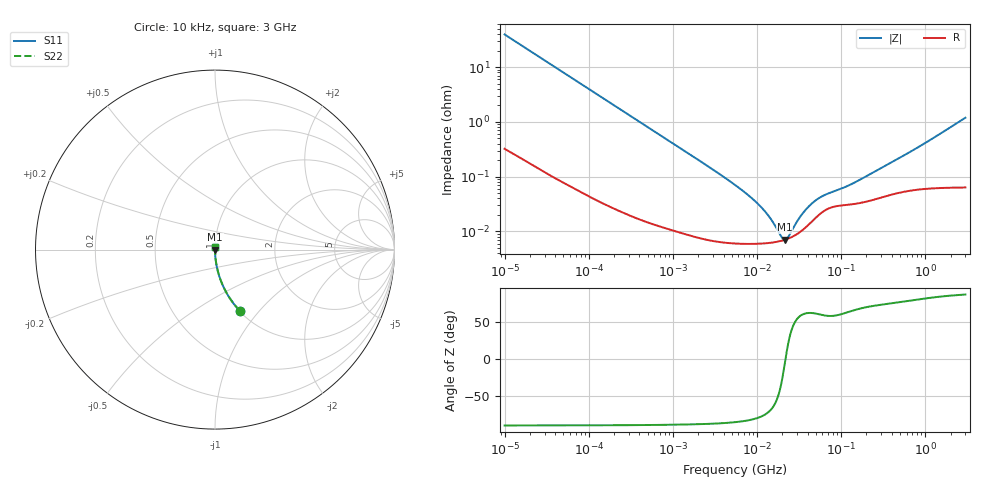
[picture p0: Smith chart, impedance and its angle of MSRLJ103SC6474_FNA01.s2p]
! MSRLJ103SC6474_FNA01  S-PARAMETER MODEL  ( Standard Model )
! Model Generated by TAIYO YUDEN Corporation (http://www.ty-top.com)
! Version 1.0
! TAIYO YUDEN Control No. 220601
! Copyright(c) 2010 TAIYO YUDEN CO.,LTD. All Rights Reserved.
! Product Description (link to TY-COMPAS)
! https://ds.yuden.co.jp/TYCOMPAS/or/detail?pn=MSRLJ103SC6474MFNA01&u=M
! Products Name : Multilayer Ceramic Capacitors
! Characteristics :
!  Capacitance : 0.47 [uF] , Rated Voltage : 6.3 [V] , TCC : X6S
!  Case Size : 0.52 x 1.0 / 0.02 x 0.039 [mm/inch] , Thickness : 0.3 / 0.012 [mm/inch]
!  (Conditions: Temperature = 25 [degC] , DC Bias Voltage = 0 [V])
! External Node Assignments :
!  1  o---| |---o  2
! GND o---------o GND
! Frequency Range : 10kHz  -  3GHz  [ 401 STEP ]
# MHZ S RI R 50
! Freq[MHz].  S11 Real  S11 Imag  S21 Real  S21 Imag  S12 Real  S12 Imag  S22 Real  S22 Imag
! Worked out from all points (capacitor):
!   401 points, 10 kHz to 3 GHz, reference 50 ohm
!   read as one part in series: C = 403 nF near 10.65 kHz
!   lowest |Z| = 7.06 mohm at 21.25 MHz (marker M1)
!   series resonance near 21.82 MHz, so ESL is about 130 pH
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0.01  0.1366 -0.3393  0.8634 0.3393  0.8634 0.3393  0.1366 -0.3393
0.016047  0.059 -0.2313  0.941 0.2313  0.941 0.2313  0.059 -0.2313
0.027426  0.0217 -0.1412  0.9783 0.1412  0.9783 0.1412  0.0217 -0.1412
0.082683  0.00283 -0.0481  0.9972 0.0481  0.9972 0.0481  0.00283 -0.0481
0.683653  0.000159 -0.00591  0.9998 0.00591  0.9998 0.00591  0.000159 -0.00591
2.652321  7.14e-05 -0.00152  0.9999 0.00152  0.9999 0.00152  7.14e-05 -0.00152
5.477226  6.05e-05 -0.000703  0.9999 0.000703  0.9999 0.000703  6.05e-05 -0.000703
8.252149  5.92e-05 -0.000428  0.9999 0.000428  0.9999 0.000428  5.92e-05 -0.000428
10.95979  5.98e-05 -0.000282  0.9999 0.000282  0.9999 0.000282  5.98e-05 -0.000282
13.66633  6.13e-05 -0.000184  0.9999 0.000184  0.9999 0.000184  6.13e-05 -0.000184
17.5871  6.5e-05 -8.27e-05  0.9999 8.27e-05  0.9999 8.27e-05  6.5e-05 -8.27e-05
18.73182  6.63e-05 -5.84e-05  0.9999 5.84e-05  0.9999 5.84e-05  6.63e-05 -5.84e-05
21.24962  6.99e-05 -1.01e-05  0.9999 1.01e-05  0.9999 1.01e-05  6.99e-05 -1.01e-05
24.10585  7.5e-05 3.82e-05  0.9999 -3.82e-05  0.9999 -3.82e-05  7.5e-05 3.82e-05
25.67485  7.83e-05 6.25e-05  0.9999 -6.25e-05  0.9999 -6.25e-05  7.83e-05 6.25e-05
35.19136  0.000107 0.000188  0.9999 -0.000188  0.9999 -0.000188  0.000107 0.000188
45.28751  0.000154 0.000289  0.9998 -0.000289  0.9998 -0.000289  0.000154 0.000289
60.14696  0.000226 0.00038  0.9998 -0.00038  0.9998 -0.00038  0.000226 0.00038
132.292  0.000312 0.000658  0.9997 -0.000658  0.9997 -0.000658  0.000312 0.000658
374.4521  0.00046 0.00167  0.9995 -0.00167  0.9995 -0.00167  0.00046 0.00167
877.2067  0.000598 0.0036  0.9994 -0.0036  0.9994 -0.0036  0.000598 0.0036
3000  0.000775 0.0119  0.9992 -0.0119  0.9992 -0.0119  0.000775 0.0119
